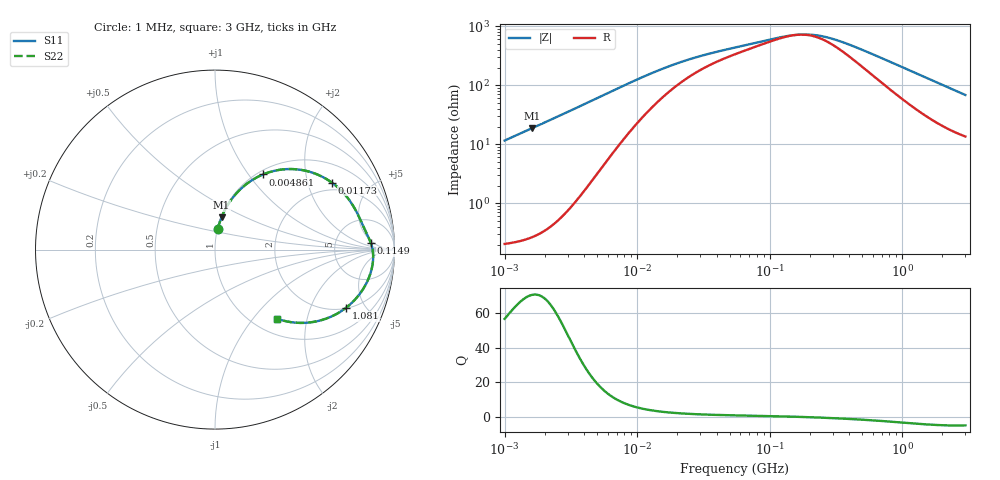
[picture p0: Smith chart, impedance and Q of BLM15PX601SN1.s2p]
! BLM15PX601SN1
# Hz S RI R 50
!Freq.(Hz) S11(Real) S11(Imag) S21(Real) S21(Imag) S12(Real) S12(Imag) S22(Real) S22(Imag)
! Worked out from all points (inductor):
!   401 points, 1 MHz to 3 GHz, reference 50 ohm
!   read as one part in series: L = 1.85 uH near 1.041 MHz
!   highest Q = 70.5 at 1.617 MHz (marker M1), where L = 1.85 uH
!   self-resonance near 162 MHz
!   S11 on the Smith chart (normalised r, x): 1 MHz: 1.00, +0.23; 4.861 MHz: 1.06, +1.18; 11.73 MHz: 1.67, +2.86; 114.9 MHz: 13, +4; 1.081 GHz: 2.03, -3.63; 3 GHz: 1.27, -1.34
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1000000  0.0152 0.1138  0.9848 -0.1138  0.9848 -0.1138  0.0152 0.1138
1616692  0.0365 0.1807  0.9635 -0.1807  0.9635 -0.1807  0.0365 0.1807
2613693  0.0904 0.278  0.9096 -0.278  0.9096 -0.278  0.0904 0.278
3823119  0.1804 0.3691  0.8196 -0.3691  0.8196 -0.3691  0.1804 0.3691
4861065  0.2678 0.4188  0.7322 -0.4188  0.7322 -0.4188  0.2678 0.4188
6058321  0.3665 0.4454  0.6335 -0.4454  0.6335 -0.4454  0.3665 0.4454
7400828  0.4628 0.4464  0.5372 -0.4464  0.5372 -0.4464  0.4628 0.4464
1.172775e7  0.6513 0.3732  0.3487 -0.3732  0.3487 -0.3732  0.6513 0.3732
1.461624e7  0.7109 0.3209  0.2891 -0.3209  0.2891 -0.3209  0.7109 0.3209
2.41077e7  0.7871 0.2131  0.2129 -0.2131  0.2129 -0.2131  0.7871 0.2131
5.477226e7  0.8375 0.1041  0.1625 -0.1041  0.1625 -0.1041  0.8375 0.1041
1.148668e8  0.8685 0.0357  0.1315 -0.0357  0.1315 -0.0357  0.8685 0.0357
1.582265e8  0.8775 0.00257  0.1225 -0.00257  0.1225 -0.00257  0.8775 0.00257
2.094008e8  0.8811 -0.0299  0.1189 0.0299  0.1189 0.0299  0.8811 -0.0299
2.609752e8  0.8806 -0.0583  0.1194 0.0583  0.1194 0.0583  0.8806 -0.0583
3.318279e8  0.8761 -0.0928  0.1239 0.0928  0.1239 0.0928  0.8761 -0.0928
5.364635e8  0.849 -0.176  0.151 0.176  0.151 0.176  0.849 -0.176
8.005644e8  0.7963 -0.2599  0.2037 0.2599  0.2037 0.2599  0.7963 -0.2599
1.080907e9  0.7288 -0.3251  0.2712 0.3251  0.2712 0.3251  0.7288 -0.3251
1.855641e9  0.5402 -0.4043  0.4598 0.4043  0.4598 0.4043  0.5402 -0.4043
2.312676e9  0.4495 -0.4072  0.5505 0.4072  0.5505 0.4072  0.4495 -0.4072
3e9  0.3474 -0.3858  0.6526 0.3858  0.6526 0.3858  0.3474 -0.3858
